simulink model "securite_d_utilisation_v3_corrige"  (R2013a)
settings: Solver=ode45  StartTime=0.0  StopTime=inf  RelTol=1e-3

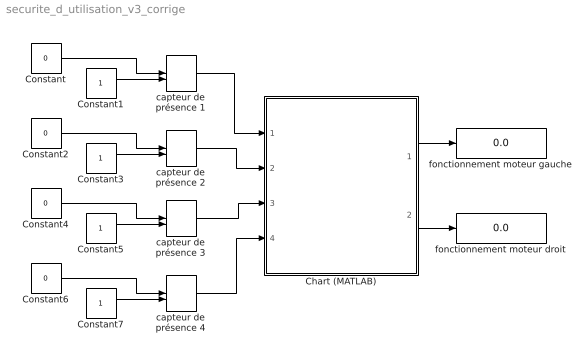
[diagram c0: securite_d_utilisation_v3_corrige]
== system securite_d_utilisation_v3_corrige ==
  Chart (MATLAB) : Stateflow chart  TreatAsAtomicUnit=on
  Constant{,2,4,6} (4 alike) : Constant  Value=0
  Constant{1,3,5,7} (4 alike) : Constant
  capteur de présence {1..4} (4 alike) : ManualSwitch
  fonctionnement moteur droit : Display
  fonctionnement moteur gauche : Display
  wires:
  Chart (MATLAB)/1(mg) -> fonctionnement moteur gauche/1
  Chart (MATLAB)/2(md) -> fonctionnement moteur droit/1
  capteur de présence 1/1 -> Chart (MATLAB)/1(p1)
  Constant1/1 -> capteur de présence 1/2
  Constant/1 -> capteur de présence 1/1
  capteur de présence 2/1 -> Chart (MATLAB)/2(p2)
  capteur de présence 3/1 -> Chart (MATLAB)/3(p3)
  capteur de présence 4/1 -> Chart (MATLAB)/4(p4)
  Constant3/1 -> capteur de présence 2/2
  Constant2/1 -> capteur de présence 2/1
  Constant5/1 -> capteur de présence 3/2
  Constant4/1 -> capteur de présence 3/1
  Constant7/1 -> capteur de présence 4/2
  Constant6/1 -> capteur de présence 4/1
